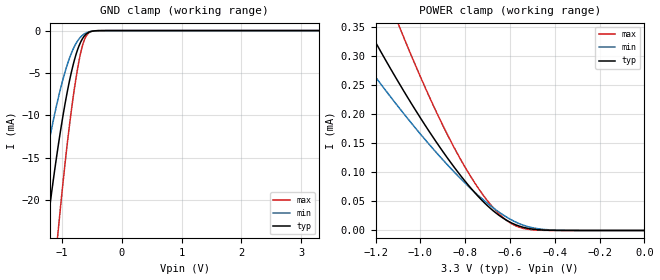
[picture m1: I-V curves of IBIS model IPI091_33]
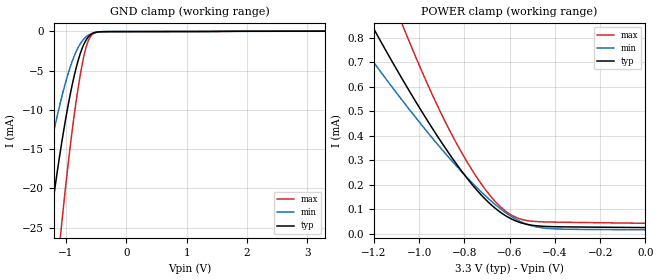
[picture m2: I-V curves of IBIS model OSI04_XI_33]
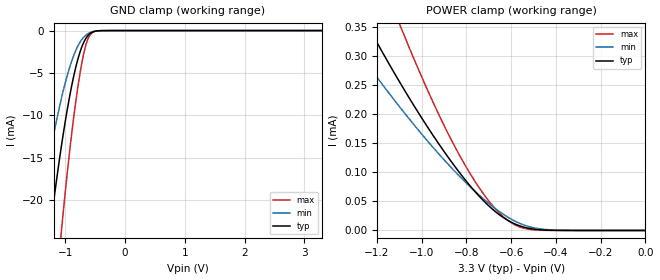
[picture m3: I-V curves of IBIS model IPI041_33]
| TEXAS INSTRUMENTS INCORPORATED
| Connectivity Solutions Group
| IBIS Model of TL16C550DZQS_3.3V
| 550D_ZQS_3.3V
| This file contains package information for the following:
|  ZQS 24-pin (BGA) package as [Component] 550DZQS_3.3V
| This device can be powered at the following Vccs:
|  3.3 Volt Vcc
| This file provides unique models under the [Model Selector] for each Vcc.
| For operation at a specific Vcc, select the appropriate model after each
| [Model Selector] keyword.
[IBIS Ver]   3.2
[Comment char]  |_char
[File Name]   550D_ZQS_3.3V.ibs
[File Rev]   1 | a
[Date]   December 15, 2008
[Source]   Data created from TI-SPICE simulations at TI-CONN.
[Notes]   The following is an IBIS list for the 550D_ZQS_3.3V.
   Please contact s-ly@ti.com with questions and
   comments concerning CONN IBIS models.
[Disclaimer] Property of Texas Instruments Incorporated.  Unauthorized
   reproduction and/or distribution is strictly prohibited.
   This product is protected under copyright law.
   Created  2003, (C) Copyright  2003, Texas Instruments
   Incorporated, All Rights Reserved
   UNLESS THERE IS A SIGNED, WRITTEN AGREEMENT TO THE
   CONTRARY, TEXAS INSTRUMENTS (TI) IS PROVIDING THE IBIS
   MODELS  AND WITHOUT ANY WARRANTY, EXPRESSED OR
   IMPLIED.  TI assumes no liability for:
   1) the accuracy of the IBIS models provided to your
   company;
   2) the proper functioning of these IBIS Models in your
   design or for any resulting applications; or
   3) infringement of patents, copyrights or intellectual
   property rights resulting from your use of these IBIS
   models.
   TI provides IBIS Models as a service to our customers.
   You and your company shall not distribute, sell or give
   these models to anyone else without prior written
   permission from TI.
   TI reserves the right to make changes to our products or
   to discontinue any semiconductor product or service
   without notice, and advises our customers to obtain the
   latest version of relevant information to verify, before
   placing orders, that the information being relied on is
   current.
   Please be aware that your receipt and use of the IBIS
   information provided shall serve as acceptance of these
   terms and conditions.  If you do not accept these terms,
   you should return or destroy the IBIS models and any
   other accompanying information immediately.
| Component 550D_3.3V_ZQS 24-pin BGA
[Component]   550D_ZQS_3.3V
[Manufacturer]   Texas Instruments, Inc.
[Package]
|   typ   min   max
R_pkg   4.665e-02   3.264e-02   6.067e-02
L_pkg   1.009e-09   0.683e-09   1.336e-09
C_pkg   2.424e-13   1.463e-13   3.850e-13
[Pin]   signal_name   model_name   R_pin   L_pin   C_pin
A1   D5   IPI04_OPJ43   3.914e-02   0.909e-09   1.463e-13
A2   D4   IPI04_OPJ43   3.358e-02   0.717e-09   1.685e-13
A3   D2   IPI04_OPJ43   3.418e-02   0.721e-09   1.686e-13
A4   D0   IPI04_OPJ43   3.779e-02   0.849e-09   1.744e-13
A5   VCC   POWER   4.675e-02   1.160e-09   1.698e-13
B1   D7   IPI04_OPJ43   3.408e-02   0.733e-09   1.672e-13
B3   D3   IPI04_OPJ43   4.552e-02   0.909e-09   3.306e-13
B4   D1   IPI04_OPJ43   4.866e-02   1.034e-09   3.084e-13
B5   MR   IPI091   3.264e-02   0.686e-09   1.664e-13
C1   SIN   IPI041   3.268e-02   0.683e-09   1.584e-13
C2   SOUT   OPJ430   4.586e-02   0.916e-09   3.238e-13
C3   D6   IPI04_OPJ43   5.719e-02   1.336e-09   3.850e-13
C4   CTSB   IPI041   6.067e-02   1.225e-09   3.274e-13
C5   RTSB   OPJ430   3.287e-02   0.693e-09   1.555e-13
D1   CS2B   IPI041   3.303e-02   0.701e-09   1.630e-13
D2   WR1B   IPI041   4.588e-02   0.923e-09   2.961e-13
D3   RD1B   IPI041   4.627e-02   0.925e-09   3.222e-13
D4   INTRPT   OPJ430   4.611e-02   0.954e-09   2.955e-13
D5   A0   IPI041   3.389e-02   0.724e-09   1.619e-13
E1   XIN   OSI04_XI   3.991e-02   0.937e-09   1.534e-13
E2   XOUT   OSI04   3.400e-02   0.722e-09   1.635e-13
E3   VSS   GND   3.336e-02   0.700e-09   1.624e-13
E4   A2   IPI041   3.740e-02   0.828e-09   1.710e-13
E5   A1   IPI041   4.103e-02   0.969e-09   1.494e-13
| Model IPI091
[Model Selector]   IPI091
IPI091_33   3.3 volt Vcc
| Model OSI04_XI
[Model Selector]   OSI04_XI
OSI04_XI_33   3.3 volt Vcc
| Model IPI041
[Model Selector]   IPI041
IPI041_33   3.3 volt Vcc
| Model IPI04_OPJ43
[Model Selector]   IPI04_OPJ43
IPI04_OPJ43_33   3.3 volt Vcc
| Model OPJ430
[Model Selector]   OPJ430
OPJ430_33   3.3 volt Vcc
| Model OSI04
[Model Selector]   OSI04
OSI04_33   3.3 volt Vcc
| Models and submodels in the file (6): IPI091_33 (Input), OSI04_XI_33 (Input), IPI041_33 (Input), IPI04_OPJ43_33 (I/O), OPJ430_33 (3-state), OSI04_33 (3-state)
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[Model]   IPI091_33
Model_type  Input
Vinl = 0
Vinh = 3.3
| variable   typ   min   max
C_comp   1.07pF   0.95pF   1.20pF
[Temperature Range]   40   125   -40
| Ambient temperature   25   110   -40
[Voltage range]   3.3   3   3.6
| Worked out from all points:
|   GND clamp passes 1 mA (typ) near -0.66 V on its own axis
|   POWER clamp passes 1 mA (typ) near -2.03 V on its own axis
[GND Clamp]
| IPI091_33
|   Voltage   I(typ)   I(min)   I(max)
-3.3V     -184.1mA   -131.7mA   -253.5mA
-1.485V   -37.43mA   -23.94mA   -59.12mA
-1.28V    -24.78mA   -15.34mA   -40.66mA
-1.25V    -23.07mA   -14.2mA    -38.11mA
-1.075V   -13.97mA   -8.224mA   -24.19mA
-1.06V    -13.26mA   -7.774mA   -23.08mA
-940mV    -8.152mA   -4.58mA    -14.87mA
-805mV    -3.718mA   -2.005mA   -7.28mA
-700mV    -1.488mA   -825uA     -2.909mA
-600mV    -421.4uA   -273uA     -659.6uA
-400mV    -8.531uA   -12.92uA   -6.748uA
3.3V      251.6pA    69.15nA    65.83pA
[POWER Clamp]
| IPI091_33
|   Voltage   I(typ)   I(min)   I(max)
-3.3V     2.289mA    1.713mA    3.253mA
-1.35V    432uA      344.6uA    613.8uA
-1.225V   341.4uA    277.2uA    481uA
-1.11V    263.3uA    218.6uA    366.4uA
-1.075V   240.6uA    201.5uA    333.1uA
-930mV    152.9uA    134.7uA    205.1uA
-805mV    87.01uA    83.43uA    112uA
-700mV    42.42uA    46.59uA    50.87uA
-620mV    18.66uA    24.18uA    18.85uA
-540mV    5.375uA    9.01uA     3.55uA
-445mV    638.3nA    1.643uA    187.2nA
-47.99fV  251.6pA    2.2nA      73.1pA
[Model]   OSI04_XI_33
Model_type  Input
Vinl = 0
Vinh = 3.3
| variable   typ   min   max
C_comp   1.85pF   1.15pF   2.42pF
[Temperature Range]   40   125   -40
| Ambient temperature   25   110   -40
[Voltage range]   3.3   3   3.6
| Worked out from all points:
|   GND clamp passes 1 mA (typ) near -0.66 V on its own axis
|   POWER clamp passes 1 mA (typ) near -1.30 V on its own axis
[GND Clamp]
| OSI04_XI_33
|   Voltage   I(typ)   I(min)   I(max)
-3.3V     -187.4mA   -133.6mA   -258.6mA
-1.52V    -40.73mA   -26.12mA   -63.96mA
-1.48V    -38.05mA   -24.28mA   -60.12mA
-1.275V   -25.2mA    -15.59mA   -41.32mA
-1.095V   -15.43mA   -9.17mA    -26.46mA
-1.07V    -14.21mA   -8.387mA   -24.55mA
-935mV    -8.294mA   -4.704mA   -15.09mA
-800mV    -3.791mA   -2.104mA   -7.36mA
-695mV    -1.529mA   -912.1uA   -2.917mA
-600mV    -479.4uA   -361uA     -744.5uA
-390mV    -35.35uA   -32.95uA   -52.71uA
3.3V      25.17uA    17.8uA     39.06uA
[POWER Clamp]
| OSI04_XI_33
|   Voltage   I(typ)   I(min)   I(max)
-3.3V     5.294mA    3.984mA    7.572mA
-1.3V     1.007mA    827.6uA    1.402mA
-1.195V   827.7uA    692.7uA    1.14mA
-1.075V   632.4uA    545.1uA    855.7uA
-1.04V    577.7uA    503.5uA    776.7uA
-915mV    392.6uA    361.2uA    514.8uA
-815mV    259.4uA    256uA      336.3uA
-720mV    152.9uA    166.1uA    196.6uA
-625mV    77.8uA     91.06uA    97.45uA
-555mV    46.18uA    50.98uA    60.77uA
-455mV    30.55uA    24.01uA    48.59uA
-47.99fV  25.17uA    16.02uA    42.63uA
[Model]   IPI041_33
Model_type  Input
Vinl = 0
Vinh = 3.3
| variable   typ   min   max
C_comp   1.08pF   0.95pF   1.21pF
[Temperature Range]   40   125   -40
| Ambient temperature   25   110   -40
[Voltage range]   3.3   3   3.6
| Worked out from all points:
|   GND clamp passes 1 mA (typ) near -0.66 V on its own axis
|   POWER clamp passes 1 mA (typ) near -2.03 V on its own axis
[GND Clamp]
| IPI041_33
|   Voltage   I(typ)   I(min)   I(max)
-3.3V     -184.1mA   -131.7mA   -253.5mA
-1.485V   -37.43mA   -23.94mA   -59.12mA
-1.28V    -24.78mA   -15.34mA   -40.66mA
-1.25V    -23.07mA   -14.2mA    -38.11mA
-1.075V   -13.97mA   -8.224mA   -24.19mA
-1.06V    -13.26mA   -7.774mA   -23.08mA
-940mV    -8.152mA   -4.58mA    -14.87mA
-805mV    -3.718mA   -2.005mA   -7.28mA
-700mV    -1.488mA   -825uA     -2.909mA
-600mV    -421.4uA   -273uA     -659.6uA
-400mV    -8.531uA   -12.92uA   -6.748uA
3.3V      251.6pA    69.15nA    65.83pA
[POWER Clamp]
| IPI041_33
|   Voltage   I(typ)   I(min)   I(max)
-3.3V     2.289mA    1.713mA    3.253mA
-1.35V    432uA      344.6uA    613.8uA
-1.225V   341.4uA    277.2uA    481uA
-1.11V    263.3uA    218.6uA    366.4uA
-1.075V   240.6uA    201.5uA    333.1uA
-930mV    152.9uA    134.7uA    205.1uA
-805mV    87.01uA    83.43uA    112uA
-700mV    42.42uA    46.59uA    50.87uA
-620mV    18.66uA    24.18uA    18.85uA
-540mV    5.375uA    9.01uA     3.55uA
-445mV    638.3nA    1.643uA    187.2nA
-47.99fV  251.6pA    2.2nA      73.1pA
